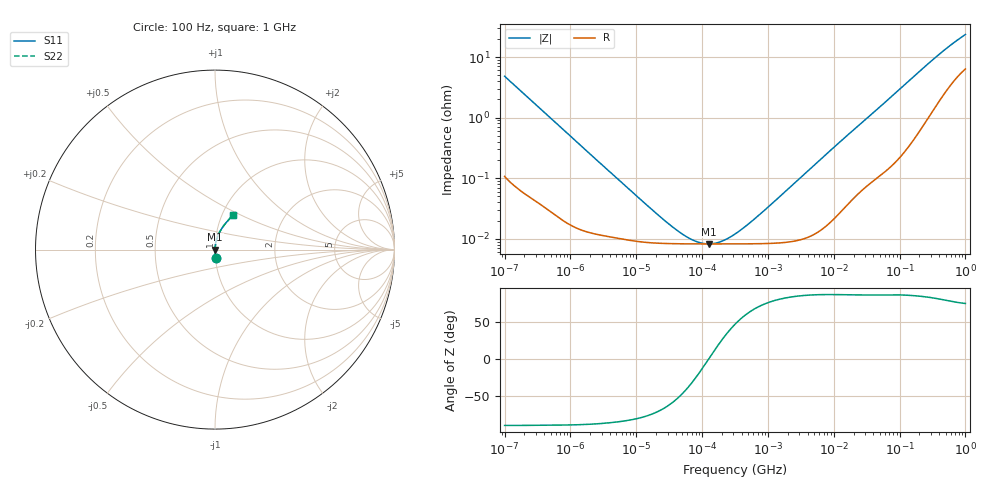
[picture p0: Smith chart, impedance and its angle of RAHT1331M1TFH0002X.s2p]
! RAHT1331M1TFH0002X  S-PARAMETER MODEL  (AEC-Q200 qualified)
! Model Generated by ELNA Corporation (http://www.ty-top.com)
! Version 1.0
! ELNA Control No. 201214
! Copyright (c) 2020 ELNA CO.,LTD. All Rights Reserved.
! Products Name : CONDUCTIVE POLYMER HYBRID ALUMINUM ELECTROLYTIC CAPACITORS
! Characteristics :
!  Capacitance  :  330uF  ,  Rated voltage  :  25V
!  Operating Temp. Range  :  -55 to +105 degC  ,  Endurance  :  5000hr at 105 degC
!  Dimension D  :  10mm  ,  Dimension L  :  10mm
! Frequency Range : 100Hz - 1GHz
! External Node Assignments :
!  1  o---| |---o  2
# MHz S RI R 50
!Freq[MHz].  S11 Real  S11 Imag  S21 Real  S21 Imag  S12 Real  S12 Imag  S22 Real  S22 Imag
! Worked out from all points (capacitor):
!   401 points, 100 Hz to 1 GHz, reference 50 ohm
!   read as one part in series: C = 329 uF near 108 Hz
!   lowest |Z| = 8.22 mohm at 125.2 kHz (marker M1)
!   series resonance near 125.7 kHz, so ESL is about 4.9 nH
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0.0001  0.00339 -0.048  0.9966 0.048  0.9966 0.048  0.00339 -0.048
0.000113  0.00275 -0.0426  0.9972 0.0426  0.9972 0.0426  0.00275 -0.0426
0.000285  0.00072 -0.0171  0.9993 0.0171  0.9993 0.0171  0.00072 -0.0171
0.001488  0.00015 -0.00334  0.9999 0.00334  0.9999 0.00334  0.00015 -0.00334
0.022131  8.44e-05 -0.000225  0.9999 0.000225  0.9999 0.000225  8.44e-05 -0.000225
0.038905  8.29e-05 -0.00012  0.9999 0.00012  0.9999 0.00012  8.29e-05 -0.00012
0.060604  8.25e-05 -6.52e-05  0.9999 6.52e-05  0.9999 6.52e-05  8.25e-05 -6.52e-05
0.071203  8.24e-05 -4.91e-05  0.9999 4.91e-05  0.9999 4.91e-05  8.24e-05 -4.91e-05
0.12517  8.22e-05 -3.3e-07  0.9999 3.3e-07  0.9999 3.3e-07  8.22e-05 -3.3e-07
0.229087  8.22e-05 5.22e-05  0.9999 -5.22e-05  0.9999 -5.22e-05  8.22e-05 5.22e-05
0.258523  8.23e-05 6.43e-05  0.9999 -6.43e-05  0.9999 -6.43e-05  8.23e-05 6.43e-05
0.316228  8.23e-05 8.68e-05  0.9999 -8.68e-05  0.9999 -8.68e-05  8.23e-05 8.68e-05
0.454465  8.25e-05 0.000137  0.9999 -0.000137  0.9999 -0.000137  8.25e-05 0.000137
0.737055  8.3e-05 0.000233  0.9999 -0.000233  0.9999 -0.000233  8.3e-05 0.000233
4.704354  0.000116 0.00153  0.9999 -0.00153  0.9999 -0.00153  0.000116 0.00153
13.4122  0.000312 0.00427  0.9997 -0.00427  0.9997 -0.00427  0.000312 0.00427
69.9842  0.0019 0.0206  0.9981 -0.0206  0.9981 -0.0206  0.0019 0.0206
176.8072  0.00739 0.0504  0.9926 -0.0504  0.9926 -0.0504  0.00739 0.0504
380.1894  0.0272 0.1001  0.9728 -0.1001  0.9728 -0.1001  0.0272 0.1001
641.9482  0.0598 0.1475  0.9402 -0.1475  0.9402 -0.1475  0.0598 0.1475
922.5714  0.0926 0.1837  0.9074 -0.1837  0.9074 -0.1837  0.0926 0.1837
1000  0.1008 0.1921  0.8992 -0.1921  0.8992 -0.1921  0.1008 0.1921
